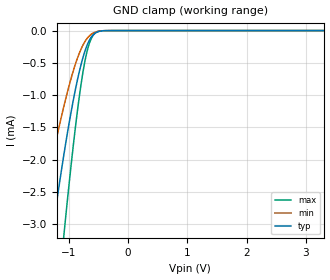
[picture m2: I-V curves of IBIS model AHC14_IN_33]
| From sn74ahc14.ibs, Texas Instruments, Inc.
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[Model]   AHC14_IN_33
Model_type  Input
Vinl=1.05
Vinh=2.34
| variable   typ   min   max
C_comp   0.56pF   0.48pF   0.64pF
[Temperature Range]   40   100   -40
| Ambient temperature   25   85   -40
[Voltage range]   3.3   3   3.6
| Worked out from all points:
|   GND clamp passes 1 mA (typ) near -0.91 V on its own axis
[GND Clamp]
| AHC14_IN_33
|   Voltage   I(typ)   I(min)   I(max)
-3.3V     -21.05mA   -13.81mA   -28.56mA
-1.52V    -4.845mA   -3.102mA   -7.626mA
-1.28V    -3.152mA   -1.986mA   -5.103mA
-1.1V     -2.026mA   -1.242mA   -3.338mA
-1.07V    -1.853mA   -1.127mA   -3.059mA
-905mV    -992.8uA   -569.2uA   -1.634mA
-835mV    -688.4uA   -381.4uA   -1.112mA
-770mV    -449.4uA   -241.9uA   -697.8uA
-675mV    -193uA     -104uA     -265.5uA
-575mV    -52.68uA   -32.07uA   -58.38uA
-375mV    -1.402uA   -1.027uA   -717.1nA
3.3V      3.885nA    645.3pA    18.64nA
